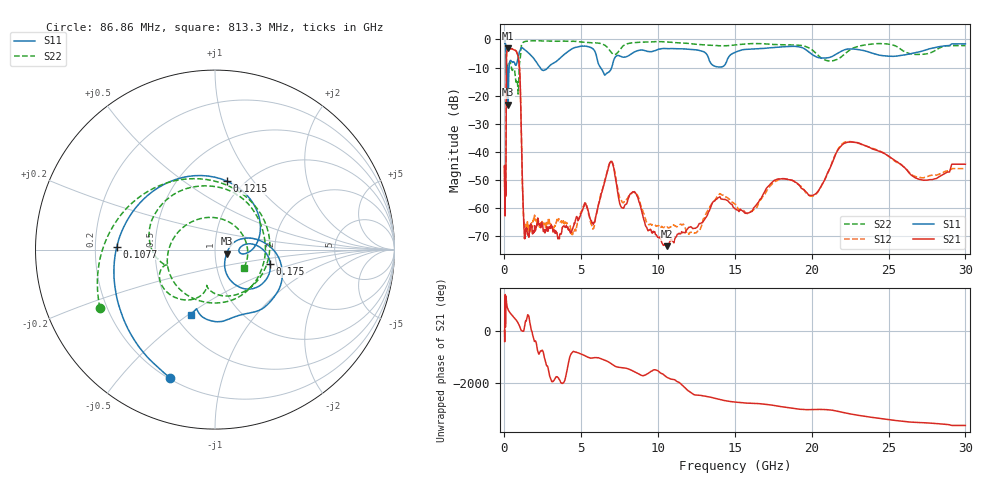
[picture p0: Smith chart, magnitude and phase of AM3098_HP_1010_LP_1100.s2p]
! Date/Time: Thu, Feb 28, 2019 8:42 AM
! Network Analyzer: Agilent Technologies E8364B Rev: A.07.50.67
! Sweep from 0.010 to 30.000 GHz, 1601 Points, Sweep Type: LOG
! Power Supply: 5.022 V, 0.002 A
# Hz S DB R 50
!freq MagS11 AngS11 MagS21 AngS21 MagS12 AngS12 MagS22 AngS22
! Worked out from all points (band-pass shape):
!   1601 points, 10 MHz to 30 GHz, reference 50 ohm
!   highest |S21| = -3.08 dB at 252.2 MHz (marker M1); lowest = -73.7 dB at 10.59 GHz (marker M2)
!   |S21| within 3 dB of the highest: 133.8 MHz to 886.6 MHz (752.7 MHz wide, 148 % of centre)
!   lowest |S11| = -23.2 dB at 241.1 MHz (marker M3), VSWR 1.15, Z = 56.9 - j2.62 ohm
!   |S11| at or under -10 dB: 192.5 MHz to 302.7 MHz (110.2 MHz wide, 44.5 % of centre); 2.323 GHz to 2.835 GHz (512.2 MHz wide, 19.9 % of centre); 6.252 GHz to 6.98 GHz (728.7 MHz wide, 11 % of centre)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
!   |S22| runs from -19.5 to -0.5 dB; largest |S21 - S12| = 0.01
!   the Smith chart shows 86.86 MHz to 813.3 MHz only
!   S11 on the Smith chart (normalised r, x): 86.86 MHz: 0.21, -0.69; 107.7 MHz: 0.29, +0.01; 121.5 MHz: 0.83, +0.75; 175 MHz: 1.85, -0.34; 813.3 MHz: 0.60, -0.51
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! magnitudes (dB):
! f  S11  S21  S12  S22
! 10 MHz  -0.4  -45.4  -46.3  -0.6
! 38.04 MHz  -0.4  -60.3  -61.3  -0.9
! 49.1 MHz  -0.7  -47.3  -51.8  -1.2
! 86.86 MHz  -2.4  -54.7  -53.8  -2.9
! 107.7 MHz  -5.2  -31.3  -31.2  -6.6
! 121.5 MHz  -8.2  -12.7  -12.7  -10.4
! 144.7 MHz  -17.5  -4.7  -4.6  -13.6
! 175 MHz  -9.9  -3.8  -3.8  -9.2
! 241.1 MHz  -23.2  -3.1  -3.1  -11.0
! 252.2 MHz  -20.6  -3.1  -3.0  -10.7
! 550.5 MHz  -8.0  -3.5  -3.5  -10.7
! 813.3 MHz  -8.2  -4.8  -4.7  -14.4
! 1.009 GHz  -4.1  -13.0  -13.0  -7.6
! 1.302 GHz  -3.6  -70.9  -65.6  -0.8
! 2.084 GHz  -8.1  -66.7  -64.4  -0.5
! 5.754 GHz  -3.3  -65.4  -67.7  -1.2
! 6.89 GHz  -11.0  -43.7  -43.5  -4.2
! 7.926 GHz  -6.2  -58.7  -57.4  -1.6
! 10.59 GHz  -3.2  -73.7  -66.8  -0.9
! 20.1 GHz  -5.6  -55.5  -55.8  -4.1
! 22.56 GHz  -3.4  -36.6  -36.4  -3.5
! 30 GHz  -1.6  -44.5  -46.0  -2.2
